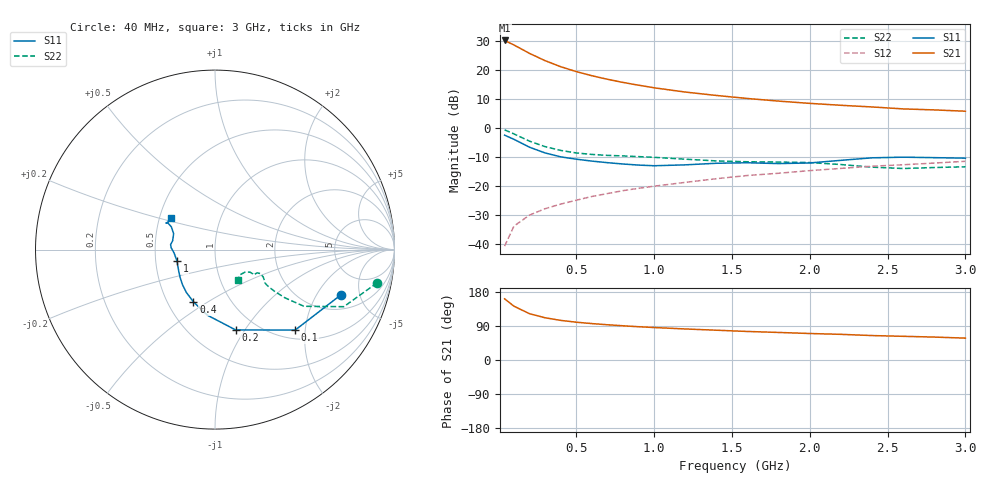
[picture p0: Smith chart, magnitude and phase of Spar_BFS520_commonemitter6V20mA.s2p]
! Filename:  BFS520K.S2P  Version:  4.0
! NXP part #: BFS520  Date: Jun 1994
! Bias condition: Vce=6V, Ic=20mA
#  MHz  S  MA  R  50
! Freq  S11  S21  S12  S22  !GUM [dB]
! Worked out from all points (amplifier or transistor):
!   21 points, 40 MHz to 3 GHz, reference 50 ohm
!   highest |S21| = 30.2 dB at 40 MHz (marker M1)
!   |S21| within 3 dB of that: start of sweep to 149.5 MHz
!   unconditionally stable (mu >= 1): 697.8 MHz to end of sweep
!   at 300 MHz: K = 0.77, MSG = 25.6 dB, |S12| = -28.0 dB
!   at 1 GHz: K = 1.07, MAG = 15.4 dB, |S12| = -20.2 dB
!   at 3 GHz: K = 1.05, MAG = 7.2 dB, |S12| = -11.6 dB
!   lowest NFmin = 1.45 dB at 500 MHz
!   S11 on the Smith chart (normalised r, x): 40 MHz: 2.92, -3.31; 100 MHz: 1.18, -1.77; 200 MHz: 0.80, -0.91; 400 MHz: 0.67, -0.43; 1 GHz: 0.65, -0.09; 3 GHz: 0.58, +0.22
40  0.746 -19.7  32.38 161.4  0.009 80.3  0.922 -11.6
100  0.633 -45.1  27.05 142.0  0.02 69.5  0.785 -23.9
200  0.462 -75.6  19.37 122.2  0.031 64.2  0.588 -32.5
300  0.368 -96.6  14.48 111.4  0.04 63.8  0.473 -34.6
400  0.315 -112.4  11.4 104.5  0.048 65.4  0.407 -35.0
500  0.287 -123.8  9.381 99.8  0.056 66.8  0.368 -34.8
600  0.266 -133.1  7.959 96.1  0.065 68.5  0.347 -34.3
700  0.25 -140.8  6.912 93.0  0.073 69.7  0.334 -33.6
800  0.237 -148.0  6.096 90.3  0.082 70.6  0.327 -32.3
900  0.227 -155.6  5.456 87.8  0.09 71.2  0.318 -31.0
1000  0.221 -162.9  4.924 85.7  0.098 71.6  0.309 -29.6
1200  0.229 -175.5  4.154 81.9  0.114 72.2  0.287 -27.8
1400  0.244 177.8  3.629 78.6  0.132 72.8  0.268 -28.9
1600  0.249 173.6  3.215 75.3  0.15 72.3  0.259 -32.3
1800  0.241 168.2  2.897 72.7  0.164 72.4  0.256 -33.3
2000  0.247 158.9  2.647 69.9  0.182 72.1  0.251 -32.7
2200  0.274 152.5  2.453 67.7  0.199 72.1  0.232 -32.8
2400  0.303 150.4  2.295 64.5  0.217 71.6  0.209 -37.0
2600  0.311 151.6  2.124 62.5  0.23 70.6  0.198 -44.8
2800  0.305 150.1  2.04 60.5  0.246 70.7  0.206 -50.3
3000  0.299 144.4  1.937 57.7  0.264 69.9  0.212 -51.9
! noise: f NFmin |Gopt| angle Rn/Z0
500  1.45  0.154  28  0.25
900  1.6  0.13  63  0.25
2000  2.2  0.228  -175  0.18
